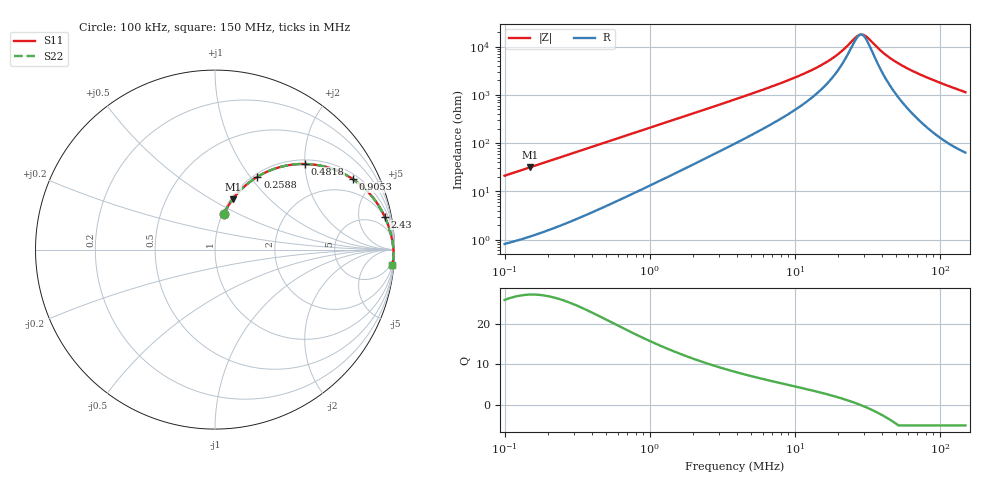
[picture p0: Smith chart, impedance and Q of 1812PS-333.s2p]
# MHz S MA R 50
!Freq  MagS11  AngS11  MagS21  AngS21  MagS12  AngS12  MagS22  AngS22
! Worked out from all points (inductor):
!   801 points, 100 kHz to 150 MHz, reference 50 ohm
!   read as one part in series: L = 33.6 uH near 103.7 kHz
!   highest Q = 27.1 at 149.5 kHz (marker M1), where L = 33.6 uH
!   self-resonance near 28.51 MHz
!   S11 on the Smith chart (normalised r, x): 100 kHz: 1.02, +0.42; 258.8 kHz: 1.04, +1.09; 481.8 kHz: 1.09, +2.01; 905.3 kHz: 1.23, +3.75; 2.43 MHz: 2, +10; 150 MHz: 2, -23
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0.1  0.2056 75.9  0.9707 -11.9  0.9707 -11.9  0.2056 75.9
0.1495151  0.2977 70.6  0.9437 -17.3  0.9437 -17.3  0.2977 70.6
0.2587569  0.4698 59.8  0.8646 -28.0  0.8646 -28.0  0.4698 59.8
0.3404045  0.5694 52.9  0.7986 -34.7  0.7986 -34.7  0.5694 52.9
0.481792  0.6932 43.5  0.6889 -43.8  0.6889 -43.8  0.6932 43.5
0.6455104  0.7829 35.6  0.5823 -51.4  0.5823 -51.4  0.7829 35.6
0.9053104  0.8615 27.2  0.4581 -59.3  0.4581 -59.3  0.8615 27.2
1.148208  0.9005 22.2  0.3783 -64.0  0.3783 -64.0  0.9005 22.2
2.429796  0.9631 11.0  0.1918 -73.5  0.1918 -73.5  0.9631 11.0
3.872983  0.9779 6.9  0.1216 -76.1  0.1216 -76.1  0.9779 6.9
8.121287  0.9882 3.1  0.05571 -76.2  0.05571 -76.2  0.9882 3.1
13.18381  0.9915 1.7  0.03017 -72.7  0.03017 -72.7  0.9915 1.7
18.83109  0.9931 0.8  0.01616 -64.2  0.01616 -64.2  0.9931 0.8
21.79702  0.9936 0.5  0.0113 -55.2  0.0113 -55.2  0.9936 0.5
26.41007  0.9942 0.2  0.006388 -24.3  0.006388 -24.3  0.9942 0.2
28.41388  0.9944 0.0  0.005626 -1.2  0.005626 -1.2  0.9944 0.0
31.13376  0.9946 -0.2  0.006189 29.1  0.006189 29.1  0.9946 -0.2
38.41884  0.995 -0.6  0.01153 64.1  0.01153 64.1  0.995 -0.6
44.46989  0.9952 -0.9  0.01651 72.7  0.01651 72.7  0.9952 -0.9
54.87553  0.9954 -1.4  0.02463 78.5  0.02463 78.5  0.9954 -1.4
71.53392  0.9953 -2.1  0.03666 81.5  0.03666 81.5  0.9953 -2.1
150  0.9913 -5.0  0.08737 81.8  0.08737 81.8  0.9913 -5.0
